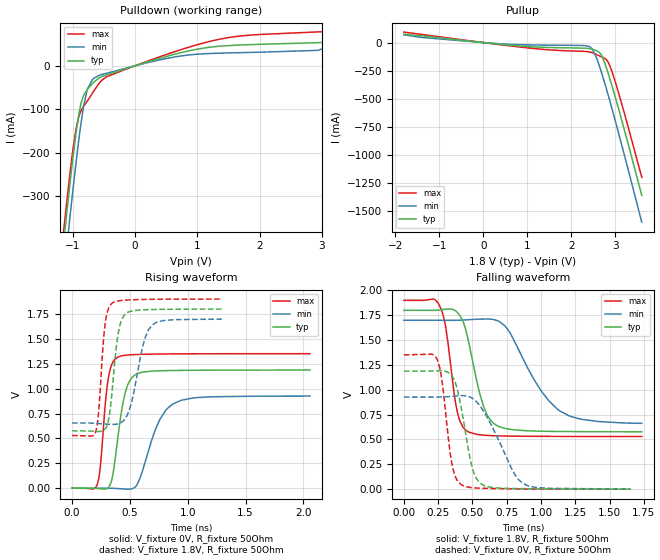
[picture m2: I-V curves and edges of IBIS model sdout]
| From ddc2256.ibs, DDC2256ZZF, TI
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|   sdout Model
[Model]   sdout
Model_type   Output
Polarity   Non-Inverting
Vmeas = 0.9
Vref = 0
Cref = 2pF
Rref = 50
|   typ   min   max
|   (nom PVT)   (fast PVT)   (slow PVT)
C_comp   2.539e-12   2.523e-12   2.572e-12
| Where nom  PVT is Nominal Process, 1.8V, 27C
|   Fast PVT is Strong Process,  1.9V, 0C
|   Slow PVT is Weak Process,   1.7V, 85C
[Voltage Range]   1.8   1.7   1.9
|Junction Temperature
[Temperature Range]   27   85   0
[Pullup Reference]   1.8   1.7   1.9
[Pulldown Reference]   0   0   0
[Power Clamp Reference]   1.8   1.7   1.9
[GND Clamp Reference]   0   0   0
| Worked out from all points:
|   slope of the pulldown table from 0 to 0.27 V, typ, clamps not added: 22.5 ohm
|   slope of the pullup table from 0 to 0.27 V, typ, clamps not added: 24.7 ohm
|   falling waveform, V_fixture 1.8V, R_fixture 50Ohm: 20-80 % time 125ps typ, 267ps min, 79.9ps max; typ from 1.8 V to 0.578 V
|   rising waveform, V_fixture 0V, R_fixture 50Ohm: 20-80 % time 91.8ps typ, 175ps min, 61.8ps max; typ from 0 V to 1.19 V
|   rising waveform, V_fixture 1.8V, R_fixture 50Ohm: 20-80 % time 67ps typ, 113ps min, 51.3ps max; typ from 0.577 V to 1.8 V
|   falling waveform, V_fixture 0V, R_fixture 50Ohm: 20-80 % time 95.8ps typ, 194ps min, 69.8ps max; typ from 1.19 V to 0.001 V
[Pulldown]
|   Voltage   I(typ)   I(min)   I(max)
-1.8V     -1.365A    -1.443A    -1.341A
-1.138V   -398.6mA   -478mA     -371.4mA
-1.046V   -275.4mA   -352.7mA   -251.6mA
-946.8mV  -156.8mA   -225.4mA   -147mA
-861.4mV  -84.62mA   -128.6mA   -102.6mA
-763mV    -54.1mA    -53.5mA    -80.91mA
-660mV    -37.56mA   -28.5mA    -57.93mA
-454.8mV  -20.59mA   -16.97mA   -25.17mA
549mV     23.46mA    18.21mA    28.44mA
1.225V    43.44mA    28.61mA    57.23mA
2.941V    53.48mA    35.82mA    78.38mA
3.6V      69.41mA    73.48mA    85.13mA
[Pullup]
|   Voltage   I(typ)   I(min)   I(max)
-1.8V     73.47mA    67.46mA    92.7mA
-1.392V   59.24mA    44.97mA    71.9mA
744.1mV   -28.24mA   -18.17mA   -36.17mA
2.29V     -49.87mA   -26.52mA   -78.77mA
2.446V    -57.34mA   -45.91mA   -87.09mA
2.561V    -70.93mA   -125.1mA   -105mA
2.664V    -100.8mA   -241.5mA   -123.5mA
2.707V    -132mA     -295.5mA   -130.3mA
2.794V    -222.6mA   -409.9mA   -151.9mA
2.876V    -323.9mA   -522.4mA   -209.3mA
3.065V    -580.2mA   -795.3mA   -438.7mA
3.6V      -1.359A    -1.596A    -1.197A
[Ramp]
R_load = 50
|   typ   min   max
dV/dt_r   0.712381/9.13221e-11   0.556166/1.72686e-10   0.810768/6.14256e-11
dV/dt_f   0.733864/1.23966e-10   0.626815/2.67976e-10   0.822167/7.97936e-11
[Falling Waveform]
V_fixture = 1.8V
V_fixture_min = 1.7V
V_fixture_max = 1.9V
R_fixture = 50Ohm
|   Time   V(typ)   V(min)   V(max)
0s        1.8V       1.7V       1.9V
214.3ps   1.799V     1.7V       1.913V
267.3ps   1.805V     1.7V       1.824V
305.5ps   1.811V     1.699V     1.627V
388.5ps   1.78V      1.699V     783.2mV
470.2ps   1.492V     1.705V     576.6mV
579.5ps   838.2mV    1.712V     543.8mV
674.5ps   643.4mV    1.699V     537mV
1.134ns   580.6mV    789.8mV    530.8mV
1.735ns   577.6mV    662.1mV    529.9mV
[Rising Waveform]
V_fixture = 0V
V_fixture_min = 0V
V_fixture_max = 0V
R_fixture = 50Ohm
|   Time   V(typ)   V(min)   V(max)
0s        234.3pV    284.5pV    353.9pV
216.3ps   -1.875mV   404.4uV    33.8mV
243.7ps   -5.153mV   410.1uV    207.5mV
312ps     4.312mV    237.8uV    1.093V
386ps     415.9mV    -2.965mV   1.31V
467.3ps   990.9mV    -8.756mV   1.336V
566.3ps   1.152V     44.61mV    1.343V
730.1ps   1.179V     617mV      1.348V
869.9ps   1.182V     844.8mV    1.349V
2.057ns   1.187V     925.7mV    1.351V
[Rising Waveform]
V_fixture = 1.8V
V_fixture_min = 1.7V
V_fixture_max = 1.9V
R_fixture = 50Ohm
|   Time   V(typ)   V(min)   V(max)
0s        576.9mV    655.3mV    529.7mV
209.6ps   570.5mV    651.1mV    585.9mV
231.3ps   570mV      649.3mV    787.3mV
285.9ps   595.8mV    644.9mV    1.649V
342.2ps   926.2mV    641mV      1.854V
399.6ps   1.558V     647.7mV    1.882V
462.7ps   1.752V     704.4mV    1.889V
633.4ps   1.793V     1.517V     1.896V
696.5ps   1.795V     1.642V     1.897V
1.295ns   1.799V     1.699V     1.9V
[Falling Waveform]
V_fixture = 0V
V_fixture_min = 0V
V_fixture_max = 0V
R_fixture = 50Ohm
|   Time   V(typ)   V(min)   V(max)
0s        1.187V     926.9mV    1.351V
236.9ps   1.191V     926.6mV    1.32V
275.1ps   1.193V     927.8mV    1.113V
351.1ps   1.139V     933.8mV    249.1mV
424.4ps   770.6mV    941.4mV    40.61mV
501.1ps   204mV      913.1mV    14.73mV
584.9ps   35.89mV    775.5mV    8.374mV
792.3ps   6.914mV    188mV      3.439mV
869.9ps   5.207mV    56.59mV    2.573mV
1.651ns   527.3uV    1.514mV    155.5uV
